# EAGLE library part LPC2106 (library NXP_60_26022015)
Single-chip 32-bit microcontrollers; 128 kB ISP/IAP ﬂash with 16/32/64 kB RAM The UART are based on a 16/32-bit ARM7TDMI-S CPU with real-time emulation and embedded trace support, together with 128 kB of embedded high speed ﬂash memory. A 128-bit wide memory interface and a unique accelerator architecture enable 32-bit code execution at maximum clock rate. For critical code size applications, the alternative 16-bit Thumb mode reduces code by more than 30 % with minimal performance penalty. Due to their tiny size and low power consumption, these microcontrollers are ideal for applications where miniaturization is a key requirement, such as access control and point-of-sale. With a wide range of serial communications interfaces and on-chip SRAM options up to 64 kB, they are very well suited for communication gateways and protocol converters, soft modems, voice recognition and low end imaging, providing both large buffer size and high processing power. Various 32-bit timers, PWM channels, and 32 GPIO lines make these microcontrollers particularly suitable for industrial control and medical systems. Remark: Throughout the data sheet, the term LPC2104/2105/2106 will apply to devices with and without /00 and /01 sufﬁxes. Sufﬁxes will be used to differentiate devices whenever they include new features. AAL Eindhoven MK
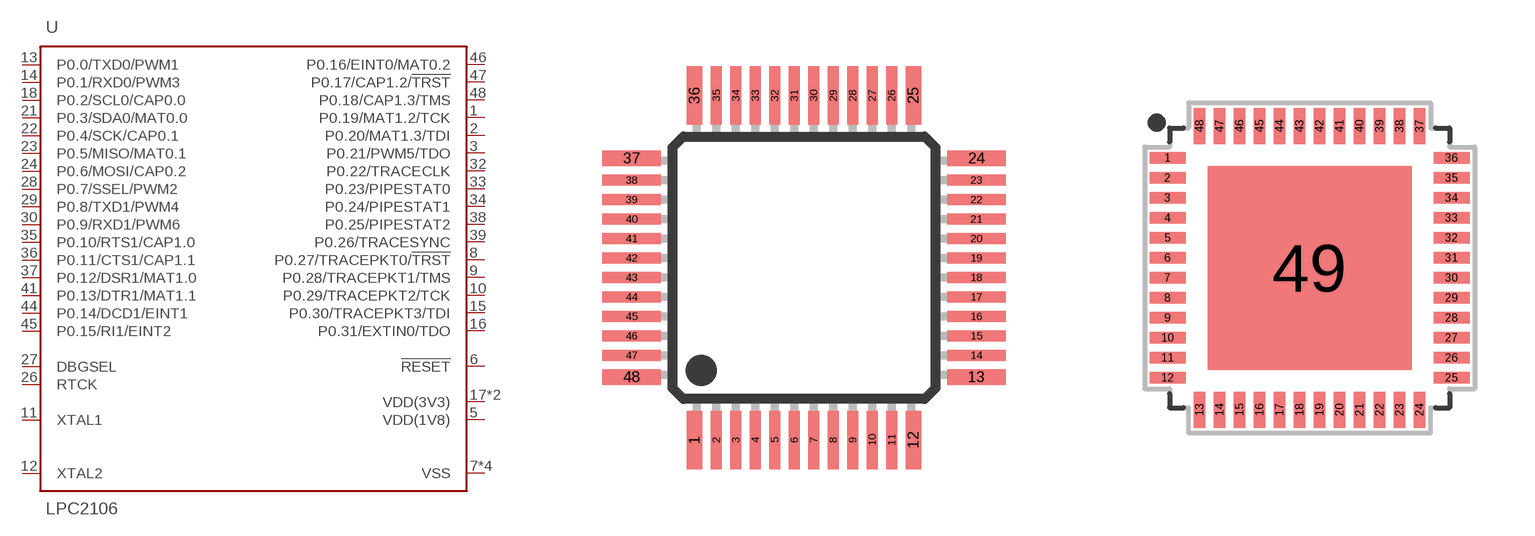
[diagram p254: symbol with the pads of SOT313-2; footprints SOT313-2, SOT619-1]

Designator prefix U

## LPC2106BBD48 (FLASH: 128kB; RANGE: 0~70C; SRAM: 64kB)  [SOT313-2]
1  P0.19/MAT1.2/TCK
2  P0.20/MAT1.3/TDI
3  P0.21/PWM5/TDO
5  VDD(1V8)  pwr
6  !RESET!
7  VSS  pwr
8  P0.27/TRACEPKT0/!TRST!
9  P0.28/TRACEPKT1/TMS
10  P0.29/TRACEPKT2/TCK
11  XTAL1
12  XTAL2
13  P0.0/TXD0/PWM1
14  P0.1/RXD0/PWM3
15  P0.30/TRACEPKT3/TDI
16  P0.31/EXTIN0/TDO
17  VDD(3V3)  pwr
18  P0.2/SCL0/CAP0.0
19  VSS  pwr
21  P0.3/SDA0/MAT0.0
22  P0.4/SCK/CAP0.1
23  P0.5/MISO/MAT0.1
24  P0.6/MOSI/CAP0.2
26  RTCK
27  DBGSEL
28  P0.7/SSEL/PWM2
29  P0.8/TXD1/PWM4
30  P0.9/RXD1/PWM6
31  VSS  pwr
32  P0.22/TRACECLK
33  P0.23/PIPESTAT0
34  P0.24/PIPESTAT1
35  P0.10/RTS1/CAP1.0
36  P0.11/CTS1/CAP1.1
37  P0.12/DSR1/MAT1.0
38  P0.25/PIPESTAT2
39  P0.26/TRACESYNC
40  VDD(3V3)  pwr
41  P0.13/DTR1/MAT1.1
43  VSS  pwr
44  P0.14/DCD1/EINT1
45  P0.15/RI1/EINT2
46  P0.16/EINT0/MAT0.2
47  P0.17/CAP1.2/!TRST!
48  P0.18/CAP1.3/TMS

## LPC2106FBD48 (FLASH: 128kB; RANGE: -40~+85C; SRAM: 64kB)  [SOT313-2]
Pads as for SOT313-2

## LPC2106FHN48 (FLASH: 128kB; RANGE: -40~+85C; SRAM: 64kB)  [SOT619-1]
Pads as for SOT313-2

## Footprint SOT313-2 (pad centres in mm)
SOT313-2 LQFP48: plastic low profile quad flat package; 48 leads; body 7 x 7 x 1.4 mm JEDEC: MS-026 IEC: 136E05 Footprint according to NXP SOT313-2 specification, however the cornerpins are 0.4mm in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
smd 0.4 x 1.5: 1 -2.81,-4.425; 12 2.81,-4.425; 25 2.81,4.425; 36 -2.81,4.425
smd 0.28 x 1.5: 2 -2.25,-4.425; 3 -1.75,-4.425; 4 -1.25,-4.425; 5 -0.75,-4.425; 6 -0.25,-4.425; 7 0.25,-4.425; 8 0.75,-4.425; 9 1.25,-4.425; 10 1.75,-4.425; 11 2.25,-4.425; 26 2.25,4.425; 27 1.75,4.425; 28 1.25,4.425; 29 0.75,4.425; 30 0.25,4.425; 31 -0.25,4.425; 32 -0.75,4.425; 33 -1.25,4.425; 34 -1.75,4.425; 35 -2.25,4.425
smd 1.5 x 0.4: 13 4.425,-2.81; 24 4.425,2.81; 37 -4.425,2.81; 48 -4.425,-2.81
smd 1.5 x 0.28: 14 4.425,-2.25; 15 4.425,-1.75; 16 4.425,-1.25; 17 4.425,-0.75; 18 4.425,-0.25; 19 4.425,0.25; 20 4.425,0.75; 21 4.425,1.25; 22 4.425,1.75; 23 4.425,2.25; 38 -4.425,2.25; 39 -4.425,1.75; 40 -4.425,1.25; 41 -4.425,0.75; 42 -4.425,0.25; 43 -4.425,-0.25; 44 -4.425,-0.75; 45 -4.425,-1.25; 46 -4.425,-1.75; 47 -4.425,-2.25

## Footprint SOT619-1 (pad centres in mm)
SOT619-1 HVQFN48: plastic thermal enhanced very thin quad flat package; no leads; 48 terminals; body 7 x 7 x 0.85 mm JEDEC: MO-220 IEC: -- JEITA: --
smd 0.9 x 0.29: 1 -3.55,2.75; 2 -3.55,2.25; 3 -3.55,1.75; 4 -3.55,1.25; 5 -3.55,0.75; 6 -3.55,0.25; 7 -3.55,-0.25; 8 -3.55,-0.75; 9 -3.55,-1.25; 10 -3.55,-1.75; 11 -3.55,-2.25; 12 -3.55,-2.75; 25 3.55,-2.75; 26 3.55,-2.25; 27 3.55,-1.75; 28 3.55,-1.25; 29 3.55,-0.75; 30 3.55,-0.25; 31 3.55,0.25; 32 3.55,0.75; 33 3.55,1.25; 34 3.55,1.75; 35 3.55,2.25; 36 3.55,2.75
smd 0.29 x 0.9: 13 -2.75,-3.55; 14 -2.25,-3.55; 15 -1.75,-3.55; 16 -1.25,-3.55; 17 -0.75,-3.55; 18 -0.25,-3.55; 19 0.25,-3.55; 20 0.75,-3.55; 21 1.25,-3.55; 22 1.75,-3.55; 23 2.25,-3.55; 24 2.75,-3.55; 37 2.75,3.55; 38 2.25,3.55; 39 1.75,3.55; 40 1.25,3.55; 41 0.75,3.55; 42 0.25,3.55; 43 -0.25,3.55; 44 -0.75,3.55; 45 -1.25,3.55; 46 -1.75,3.55; 47 -2.25,3.55; 48 -2.75,3.55
smd 5.1 x 5.1: 49 0,0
